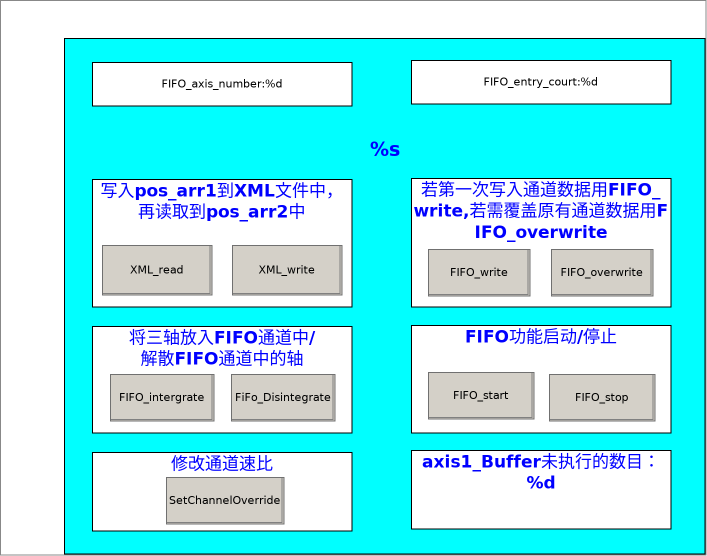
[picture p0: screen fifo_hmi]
VISUALIZATION fifo_hmi  // 707x556
    Group (64,38 641x516)
        RoundedRectangle (0,0 641x516)
        RoundedRectangle (28,24 260x44), "FIFO_axis_number:%d", text variable: MAIN.FiFo_GetDimension.iNoOfAxes
        RoundedRectangle (347,22 260x44), "FIFO_entry_court:%d", text variable: MAIN.FiFo_GetDimension.iNoOfFifoEntries
        RoundedRectangle (47,85 549x53), "%s", text variable: MAIN.fifo_display
        RoundedRectangle (28,141 260x128), "写入pos_arr1到XML文件中， 再读取到pos_arr2中"
        Button (38,207 110x50), "XML_read", colour toggle: MAIN.read_do
            tap MAIN.read_do
        Button (168,207 110x50), "XML_write", colour toggle: MAIN.writh_do
            tap MAIN.writh_do
        RoundedRectangle (28,288 260x107), "将三轴放入FIFO通道中/解散FIFO通道中的轴"
        Button (46,336 104x47), "FIFO_intergrate", colour toggle: MAIN.integrate_do
            tap MAIN.integrate_do
        Button (167,336 104x47), "FiFo_Disintegrate", colour toggle: main.FiFo_GroupDisintegrate.bExecute
            tap MAIN.FiFo_GroupDisintegrate.bExecute
        RoundedRectangle (28,414 260x79), "修改通道速比"
        Button (102,439 118x47), "SetChannelOverride", colour toggle: MAIN.FiFo_SetChannelOverride.bExecute
            tap MAIN.FiFo_SetChannelOverride.bExecute
        RoundedRectangle (347,140 260x129), "若第一次写入通道数据用FIFO_write,若需覆盖原有通道数据用FIFO_overwrite"
        Button (364,211 102x47), "FIFO_write", colour toggle: MAIN.FIFO_write_do
            tap MAIN.FIFO_write_do
        Button (487,211 102x47), "FIFO_overwrite", colour toggle: MAIN.FIFO_overwrite_do
            tap MAIN.FIFO_overwrite_do
        RoundedRectangle (347,287 260x108), "FIFO功能启动/停止"
        Button (364,334 106x47), "FIFO_start", colour toggle: MAIN.start_do
            tap MAIN.start_do
        Button (485,336 106x47), "FIFO_stop", colour toggle: MAIN.stop_do
            tap MAIN.stop_do
        RoundedRectangle (347,412 260x79), "axis1_Buffer未执行的数目： %d", text variable: MAIN.axis1.NcToPlc.SafEntries
END_VISUALIZATION
